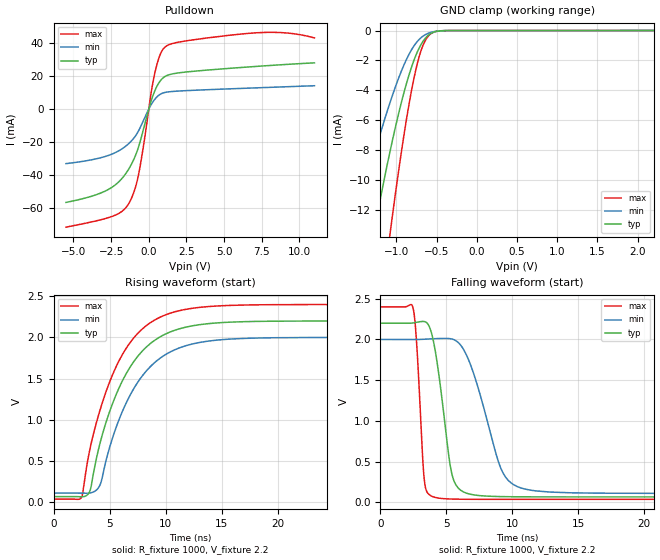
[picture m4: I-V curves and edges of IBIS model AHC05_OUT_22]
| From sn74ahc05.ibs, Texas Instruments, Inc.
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[Model]   AHC05_OUT_22
Model_type  Open_drain
Enable   Active-Low
Vref =   2.2
Rref =   1000
Cref =   50p
Vmeas =   1.1
| variable   typ   min   max
C_comp   2.30pF   1.72pF   2.62pF
| C_pulldown   4.63pF   2.55pF   7.17pF
| C_tri-state   2.30pF   1.72pF   2.62pF
[Temperature Range]   40   100   -40
| Ambient temperature   25   85   -40
[Voltage range]   2.2   2   2.4
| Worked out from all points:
|   slope of the pulldown table from 0 to 0.33 V, typ, clamps not added: 34.8 ohm
|   GND clamp passes 1 mA (typ) near -0.70 V on its own axis
|   rising waveform, R_fixture 1000, V_fixture 2.2: 20-80 % time 3.76ns typ, 3.82ns min, 3.72ns max; typ from 0.065 V to 2.2 V
|   falling waveform, R_fixture 1000, V_fixture 2.2: 20-80 % time 1.01ns typ, 1.99ns min, 463ps max; typ from 2.2 V to 0.065 V
[GND Clamp]
| AHC05_OUT_22
|   Voltage   I(typ)   I(min)   I(max)
-5.5V     -200.4mA   -131.5mA   -251.9mA
-1.55V    -22mA      -13.88mA   -34.9mA
-1.495V   -20.18mA   -12.7mA    -32.25mA
-1.285V   -13.67mA   -8.455mA   -22.45mA
-1.26V    -12.94mA   -7.982mA   -21.33mA
-1.095V   -8.459mA   -5.057mA   -14.2mA
-1.055V   -7.462mA   -4.409mA   -12.57mA
-905mV    -4.114mA   -2.279mA   -6.924mA
-780mV    -1.954mA   -1.011mA   -3.131mA
-685mV    -849uA     -438uA     -1.199mA
-580mV    -221uA     -137uA     -241.8uA
2.2V      4.508nA    1.669nA    7.99nA
[Pulldown]
| AHC05_OUT_22
|   Voltage   I(typ)   I(min)   I(max)
-5.5V     -56.5mA    -33.02mA   -71.46mA
-2.695V   -48.69mA   -28.08mA   -65.75mA
-1.81V    -42.29mA   -24.25mA   -62.08mA
-1.285V   -35.55mA   -20.48mA   -56.46mA
-930mV    -29.09mA   -16.83mA   -48.63mA
-660mV    -22.34mA   -12.81mA   -38.81mA
165mV     5.17mA     2.812mA    10.32mA
435mV     11.79mA    6.34mA     23.19mA
765mV     17.1mA     8.982mA    33.19mA
1.115V    19.93mA    10.15mA    37.84mA
7.185V    25.87mA    12.88mA    46.21mA
11V       27.99mA    14.14mA    43.1mA
[Ramp]
| AHC05_OUT_22
| variable   typ   min   max
dV/dt_r   1.28/3.76E-09   1.14/3.82E-09   1.42/3.72E-09
dV/dt_f   1.29/1.02E-09   1.14/2.01E-09   1.44/4.72E-10
R_load = 1000
[Rising Waveform]
| AHC05_OUT_22
R_fixture =   1000
C_fixture =   0
L_fixture =   0
V_fixture =   2.2
V_fixture_min = 2
V_fixture_max = 2.4
|   Time   V(typ)   V(min)   V(max)
0s        64.71mV    107.6mV    35.09mV
2.505ns   62.44mV    107.2mV    58.21mV
3.255ns   138.1mV    109.2mV    648.3mV
3.955ns   607.8mV    163.1mV    1.027V
5.23ns    1.184V     765.1mV    1.536V
6.765ns   1.625V     1.282V     1.925V
8.355ns   1.893V     1.605V     2.152V
10.25ns   2.058V     1.812V     2.287V
17.12ns   2.192V     1.988V     2.394V
50ns      2.2V       2V         2.4V
[Falling Waveform]
| AHC05_OUT_22
R_fixture =   1000
C_fixture =   0
L_fixture =   0
V_fixture =   2.2
V_fixture_min = 2
V_fixture_max = 2.4
|   Time   V(typ)   V(min)   V(max)
0s        2.2V       2V         2.4V
2.46ns    2.202V     1.999V     2.395V
2.735ns   2.211V     2V         1.984V
3.33ns    2.22V      2.003V     274.1mV
4.105ns   1.91V      2.009V     60.84mV
5.42ns    347.6mV    2.005V     38.52mV
6.745ns   100.7mV    1.727V     35.66mV
9.175ns   68.78mV    400.8mV    35.11mV
11ns      65.78mV    159.9mV    35.09mV
50ns      64.71mV    107.6mV    35.09mV
